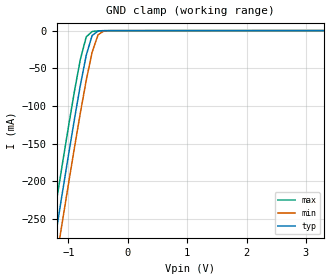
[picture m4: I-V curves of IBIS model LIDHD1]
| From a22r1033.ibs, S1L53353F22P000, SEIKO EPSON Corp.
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[Model]   LIDHD1
Model_type   Input
Polarity   Non-Inverting
Vinh=2.0V
Vinl=0.8V
|   typ   min   max
C_comp   5.0pF   4.0pF   6.0pF
|   typ   min   max
[Voltage range]   3.3   3.0   3.6
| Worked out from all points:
|   GND clamp passes 1 mA (typ) near -0.51 V on its own axis
[GND_clamp]
|   Voltage   I(typ)   I(min)   I(max)
-3.3V     -1.343A    -1.379A    -1.309A
-1.3V     -314.1mA   -352.4mA   -276.2mA
-1.2V     -264.1mA   -302.5mA   -226.1mA
-1.1V     -214.6mA   -253.1mA   -176.6mA
-1V       -165.9mA   -204.3mA   -128.1mA
-900mV    -118.4mA   -156.4mA   -81.35mA
-800mV    -73.1mA    -109.9mA   -38.61mA
-700mV    -32.76mA   -66.19mA   -8.332mA
-600mV    -6.33mA    -28.42mA   -1.141mA
-500mV    -596.9uA   -5.409mA   -249.5uA
-400mV    -64.77uA   -412.4uA   -26.72uA
3.3V      66.01uA    81.7uA     66.01uA
